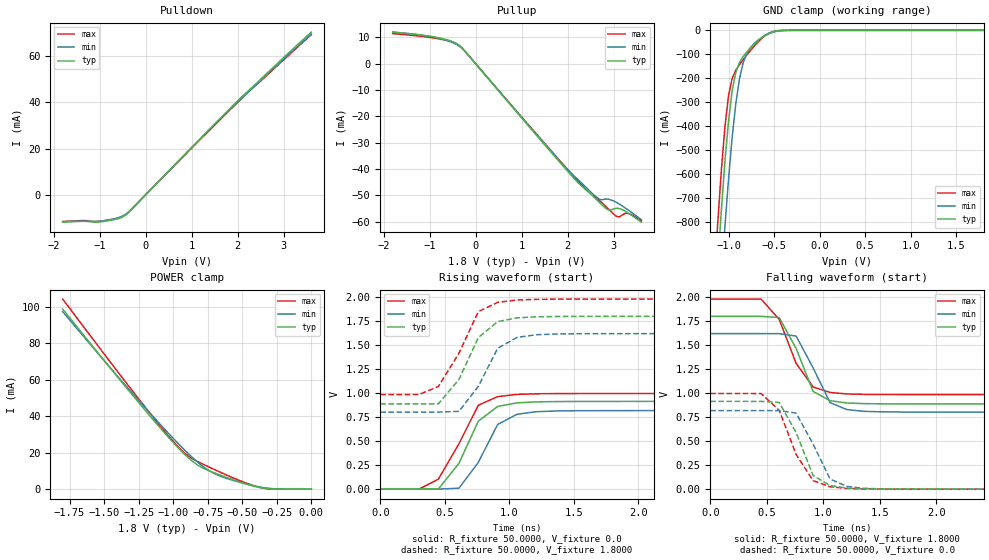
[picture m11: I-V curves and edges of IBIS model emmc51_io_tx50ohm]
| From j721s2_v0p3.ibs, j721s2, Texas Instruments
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|   Model emmc51_io_tx50ohm
[Model]  emmc51_io_tx50ohm
Model_type I/O
Polarity   Non-Inverting
Enable   Active-High
Vinl =   0.6300V
Vinh =   1.1700V
Vmeas =  0.2000V
Cref =   0.5000pF
Rref =   50.0000
Vref =   0.2000V
C_comp   2.0000pF   2.0000pF   2.0000pF
[Temperature Range]   25.0000   0.1250k   -40.0000
[Voltage Range]   1.8000V   1.6200V   1.9800V
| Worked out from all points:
|   slope of the pulldown table from 0 to 0.27 V, typ, clamps not added: 48.5 ohm
|   slope of the pullup table from 0 to 0.27 V, typ, clamps not added: 48.3 ohm
|   GND clamp passes 1 mA (typ) near -0.43 V on its own axis
|   POWER clamp passes 1 mA (typ) near -0.38 V on its own axis
|   rising waveform, R_fixture 50.0000, V_fixture 0.0: 20-80 % time 224ps typ, 207ps min, 240ps max; typ from 0 V to 0.914 V
|   rising waveform, R_fixture 50.0000, V_fixture 1.8000: 20-80 % time 231ps typ, 207ps min, 233ps max; typ from 0.888 V to 1.8 V
|   falling waveform, R_fixture 50.0000, V_fixture 1.8000: 20-80 % time 204ps typ, 211ps min, 237ps max; typ from 1.8 V to 0.888 V
|   falling waveform, R_fixture 50.0000, V_fixture 0.0: 20-80 % time 204ps typ, 212ps min, 231ps max; typ from 0.914 V to 0 V
[Pulldown]
|Voltage   I(typ)   I(min)   I(max)
-1.8V     -11.84mA   -11.66mA   -11.53mA
-1.38V    -11.49mA   -11.32mA   -11.16mA
-1.14V    -11.78mA   -11.47mA   -11.55mA
-960mV    -11.63mA   -11.36mA   -11.32mA
-600mV    -10.31mA   -9.931mA   -10.13mA
-480mV    -9.352mA   -8.971mA   -9.264mA
-420mV    -8.509mA   -8.225mA   -8.418mA
-300mV    -6.18mA    -6.105mA   -6.074mA
1.62V     33.1mA     32.78mA    32.56mA
2.22V     44.78mA    44.24mA    44.34mA
3.6V      70.46mA    69.62mA    69.33mA
[Pullup]
|Voltage   I(typ)   I(min)   I(max)
-1.8V     11.93mA    11.99mA    11.39mA
-840mV    9.937mA    9.782mA    9.536mA
-360mV    7.021mA    6.701mA    6.932mA
-180mV    3.724mA    3.671mA    3.658mA
1.92V     -39.26mA   -38.78mA   -38.62mA
2.4V      -47.91mA   -47.01mA   -47.93mA
2.7V      -52.89mA   -51.59mA   -52.13mA
2.88V     -55.54mA   -51.47mA   -55.14mA
3.06V     -54.92mA   -52.71mA   -58.01mA
3.12V     -55.04mA   -53.33mA   -58.26mA
3.3V      -56.58mA   -55.43mA   -56.86mA
3.6V      -60.23mA   -59.24mA   -59.68mA
[GND_clamp]
|Voltage   I(typ)   I(min)   I(max)
-1.8V     -6.702A    -6.906A    -6.586A
-1.12V    -991.1mA   -1.287A    -813.9mA
-1.08V    -758.6mA   -1.044A    -591.9mA
-1.04V    -552.1mA   -821.7mA   -405.1mA
-1V       -379.5mA   -621.1mA   -272.1mA
-960mV    -252.2mA   -446.8mA   -200.8mA
-920mV    -175.1mA   -305.6mA   -166.2mA
-880mV    -134mA     -202.7mA   -143.1mA
-800mV    -90.55mA   -97.27mA   -103.4mA
-600mV    -20.52mA   -21.87mA   -22.63mA
-400mV    -332.1uA   -1.109mA   -151.2uA
1.8V      231.4nA    26.73uA    254.2nA
[POWER_clamp]
|Voltage   I(typ)   I(min)   I(max)
-1.8V     98.61mA    97.2mA     104.1mA
-1.44V    64.88mA    65.13mA    68.09mA
-1.16V    39.38mA    40.99mA    40.81mA
-1V       25.58mA    27.85mA    26.18mA
-900mV    17.84mA    20.17mA    18.67mA
-820mV    13.08mA    14.63mA    15mA
-740mV    10.1mA     10.15mA    12.1mA
-660mV    7.73mA     7.169mA    9.318mA
-560mV    4.993mA    4.669mA    6.008mA
-440mV    2.128mA    2.259mA    2.491mA
-340mV    491.7uA    786.4uA    470uA
0V        231.4nA    1.21uA     740.9nA
[Ramp]
| variable   typ   min   max
dV/dt_r  0.5484/0.2206n   0.4910/0.2073n   0.5979/0.2324n
dV/dt_f  0.5474/0.2036n   0.4904/0.2107n   0.5968/0.2361n
R_load = 50.0000
[Rising Waveform]
R_fixture= 50.0000
V_fixture= 0.0
V_fixture_min= 0.0
V_fixture_max= 0.0
|time   V(typ)   V(min)   V(max)
0s        1.519uV    15.45uV    3.175uV
300ps     136uV      33.92uV    473.4uV
450ps     1.077mV    294.9uV    103.7mV
610ps     269.7mV    10.44mV    473.2mV
760ps     708.8mV    279.5mV    874.1mV
910ps     861.5mV    673.8mV    963.9mV
1.06ns    898.9mV    780.4mV    987.1mV
1.21ns    909.3mV    806.9mV    993.5mV
1.67ns    913.8mV    817.7mV    996.3mV
15ns      914mV      818.3mV    996.4mV
[Rising Waveform]
R_fixture= 50.0000
V_fixture= 1.8000
V_fixture_min= 1.6200
V_fixture_max= 1.9800
|time   V(typ)   V(min)   V(max)
0s        887.7mV    802.6mV    985.3mV
300ps     887.9mV    802.6mV    985.8mV
450ps     888.8mV    802.8mV    1.069V
610ps     1.143V     810.5mV    1.415V
760ps     1.579V     1.071V     1.849V
910ps     1.745V     1.467V     1.946V
1.06ns    1.784V     1.581V     1.97V
1.21ns    1.795V     1.608V     1.977V
1.67ns    1.8V       1.619V     1.98V
15ns      1.8V       1.62V      1.98V
[Falling Waveform]
R_fixture= 50.0000
V_fixture= 1.8000
V_fixture_min= 1.6200
V_fixture_max= 1.9800
|time   V(typ)   V(min)   V(max)
0s        1.8V       1.62V      1.98V
450ps     1.8V       1.62V      1.98V
610ps     1.788V     1.62V      1.768V
760ps     1.464V     1.594V     1.309V
910ps     1.018V     1.263V     1.065V
1.06ns    921.4mV    901.1mV    1.007V
1.21ns    897.6mV    828.6mV    991.7mV
1.36ns    891mV      810.5mV    987.4mV
1.82ns    887.9mV    803mV      985.4mV
15ns      887.7mV    802.6mV    985.3mV
[Falling Waveform]
R_fixture= 50.0000
V_fixture= 0.0
V_fixture_min= 0.0
V_fixture_max= 0.0
|time   V(typ)   V(min)   V(max)
0s        914mV      818.3mV    996.4mV
450ps     913.8mV    818.3mV    995.9mV
610ps     903.3mV    818.1mV    821.6mV
760ps     588.6mV    792mV      360.9mV
910ps     142.7mV    468.9mV    89.03mV
1.06ns    37.33mV    105.7mV    24.88mV
1.21ns    11.17mV    28.33mV    7.541mV
1.36ns    3.719mV    8.891mV    2.512mV
1.82ns    219.1uV    552.8uV    126.6uV
15ns      1.46uV     15.41uV    3.099uV
